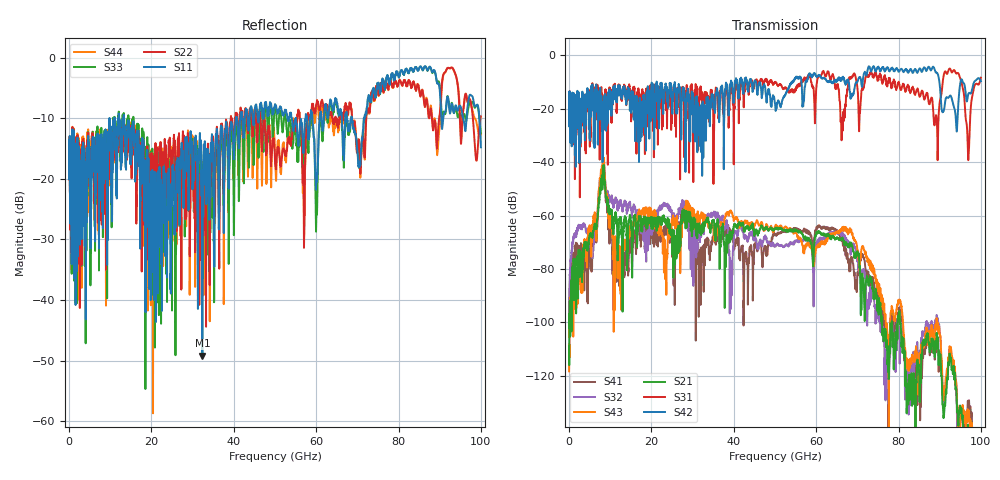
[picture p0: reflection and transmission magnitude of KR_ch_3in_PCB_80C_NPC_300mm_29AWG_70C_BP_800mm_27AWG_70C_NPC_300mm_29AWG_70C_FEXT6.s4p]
# GHz S RI R 45
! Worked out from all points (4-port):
!   4000 points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, 25 MHz to 100 GHz, reference 45 ohm
!   strongest paths, dB at 25 MHz, 25.02 GHz, 50.02 GHz, 75.03 GHz, 100 GHz:
!     S42: -20.0, -17.9, -18.0, -4.4, -9.7
!     S31: -20.0, -21.5, -10.3, -8.7, -8.4
!     S21: -109.0, -69.9, -65.0, -92.8, -174.4
!     S43: -118.3, -62.3, -64.1, -85.4, -169.2
!     S32: -98.5, -60.9, -71.5, -96.4, -182.2
!     S41: -105.5, -68.7, -67.3, -89.3, -167.5
!   lowest |S11| = -49.2 dB at 32.38 GHz (marker M1), VSWR 1.01, Z = 45.2 + j0.274 ohm
!   |S11| at or under -10 dB: start of sweep to 9.824 GHz; 13.32 GHz to 40.53 GHz (27.22 GHz wide, 101 % of centre); 68.67 GHz to 71.58 GHz (2.909 GHz wide, 4.15 % of centre)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
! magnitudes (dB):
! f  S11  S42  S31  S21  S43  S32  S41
! 25 MHz  -16.1  -20.0  -20.0  -109.0  -118.3  -98.5  -105.5
! 8.125 GHz  -14.4  -29.4  -15.9  -48.1  -42.5  -45.6  -44.3
! 12.32 GHz  -11.3  -12.8  -12.4  -61.2  -74.7  -54.7  -79.2
! 32.38 GHz  -49.2  -23.2  -21.1  -66.1  -60.5  -64.8  -75.9
! 92.53 GHz  -9.2  -15.1  -5.0  -112.9  -109.6  -111.7  -110.6
! 96.88 GHz  -7.6  -15.0  -37.6  -140.1  -134.3  -145.6  -130.7
! 100 GHz  -14.8  -9.7  -8.4  -174.4  -169.2  -182.2  -167.5
